(* Logix 5000 DataType export CM1T_DriveStatus; software revision 20.00 *)

TYPE CM1T_DriveStatus :
STRUCT
   StatusValue : SINT;   // Indicates status and error type
   StatusValue1 : SINT;   // Additional status values
   In_Position : BOOL;   // Drive is in position and ready to move
   Moving : BOOL;   // Drive is currently moving
   Disabled : BOOL;   // Drive is disabled
   Error : BOOL;   // Drive is in an error state
   MoveComplete : BOOL;   // Move Complete
   NewStartRequired : BOOL;   // New setpoint required
   HomeAchieved : BOOL;   // Home achieved
END_STRUCT
END_TYPE
